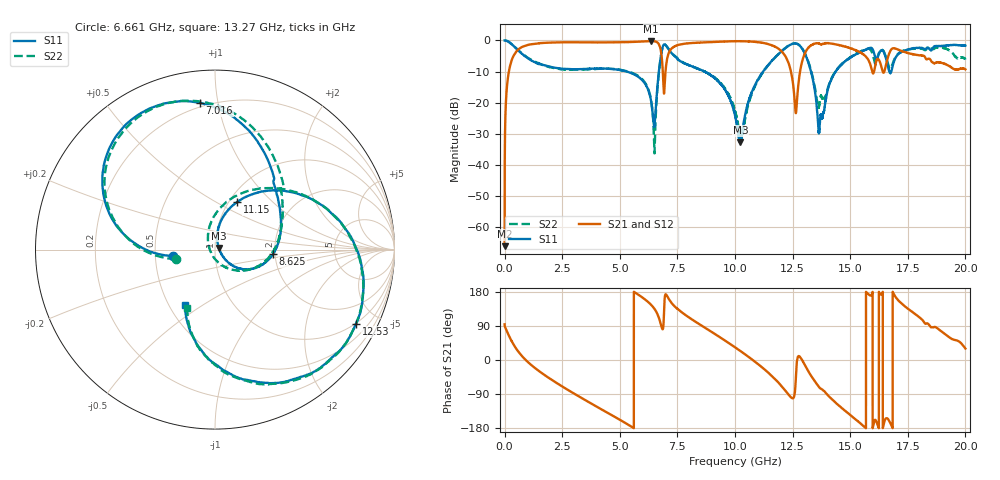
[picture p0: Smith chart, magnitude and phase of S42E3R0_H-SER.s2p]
!{S42E3R0}
!Johanson Technology Inc.
!www.johansontechnology.com
!Test Board Conditions:
!Substrate Type  RO4350B
!Substrate Thickness  50 mil
!Substrate Dk  3.66
!TL Type: GCPW
!TL Trace Width  60 mil
!TL Gap  10 mil
!Electrode orientation  Horizontal
!DUT TOPOLOGY	SERIES
!Mounting Pad LxW  14x55 mil
! Created Wed Nov 25 21:42:21 2020
# khz S ma R 50
! 2 Port Network Data from SP1.SP block
! freq  magS11  angS11  magS21  angS21  magS12  angS12  magS22  angS22
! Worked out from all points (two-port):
!   20001 points, 300 kHz to 20 GHz, reference 50 ohm
!   highest |S21| = -0.21 dB at 6.36 GHz (marker M1); lowest = -66.1 dB at 300 kHz (marker M2)
!   |S21| within 3 dB of the highest: 550.3 MHz to 6.779 GHz (6.229 GHz wide, 170 % of centre); 7.182 GHz to 11.98 GHz (4.798 GHz wide, 50.1 % of centre)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
!   lowest |S11| = -32.8 dB at 10.23 GHz (marker M3), VSWR 1.05, Z = 52.2 + j0.936 ohm
!   |S11| at or under -10 dB: 5.302 GHz to 6.696 GHz (1.394 GHz wide, 23.2 % of centre); 8.676 GHz to 11.22 GHz (2.542 GHz wide, 25.6 % of centre); 13.3 GHz to 14.37 GHz (1.067 GHz wide, 7.71 % of centre)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
!   |S22| runs from -36.3 to 0.0 dB; largest |S21 - S12| = 0.017
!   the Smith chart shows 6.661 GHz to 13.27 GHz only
!   S11 on the Smith chart (normalised r, x): 6.661 GHz: 0.62, -0.05; 7.016 GHz: 0.18, +0.89; 8.625 GHz: 1.94, -0.11; 11.15 GHz: 1.09, +0.63; 12.53 GHz: 0.98, -3.81; 13.27 GHz: 0.61, -0.42
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300  1 -0.2  0.0004945 94.2  0.0005876 85.2  0.9998 -0.3
123300  0.9744 -17.1  0.2172 72.5  0.2181 72.5  0.9748 -17.1
419300  0.7975 -52.5  0.5954 37.9  0.5963 37.9  0.8007 -52.2
1366300  0.4354 -114.4  0.8893 -23.3  0.8892 -23.3  0.4485 -113.0
3334300  0.3464 167.2  0.9356 -99.9  0.935 -99.9  0.3406 172.2
6360300  0.1048 71.6  0.9758 145.5  0.9732 145.5  0.1089 57.8
6509300  0.04333 146.5  0.9675 134.5  0.9677 134.5  0.01582 136.6
6661300  0.2382 -171.6  0.9084 117.2  0.9076 117.1  0.2235 -166.4
6667300  0.2502 -172.1  0.9016 116.3  0.9025 116.2  0.2361 -167.3
7016300  0.8218 95.8  0.4169 172.4  0.4168 172.3  0.8205 93.4
8625300  0.3229 -4.6  0.93 87.9  0.9293 88.0  0.323 -2.3
1.00003e7  0.0625 -41.6  0.9712 33.5  0.9716 33.6  0.07364 -75.5
1.02343e7  0.02297 23.0  0.9716 23.7  0.9724 23.7  0.02842 -137.1
1.11533e7  0.2918 65.2  0.9221 -18.4  0.9195 -18.4  0.2852 74.3
1.25313e7  0.8878 -27.7  0.1847 -100.7  0.1891 -100.3  0.8884 -29.2
1.32693e7  0.3484 -118.2  0.8161 -38.4  0.8143 -38.4  0.3625 -115.2
1.33343e7  0.281 -124.5  0.847 -44.7  0.8454 -44.9  0.2944 -119.1
1.36903e7  0.0516 -46.1  0.8793 -74.3  0.876 -74.1  0.111 -58.4
1.47943e7  0.4661 -45.1  0.7935 -134.7  0.7927 -134.9  0.4719 -51.3
1.66673e7  0.3475 -139.3  0.5816 -157.8  0.573 -157.9  0.3855 -141.1
1.81023e7  0.7619 -157.0  0.572 107.4  0.5795 108.9  0.731 -161.7
2e7  0.8277 133.1  0.3438 30.2  0.3457 31.0  0.4941 121.4
